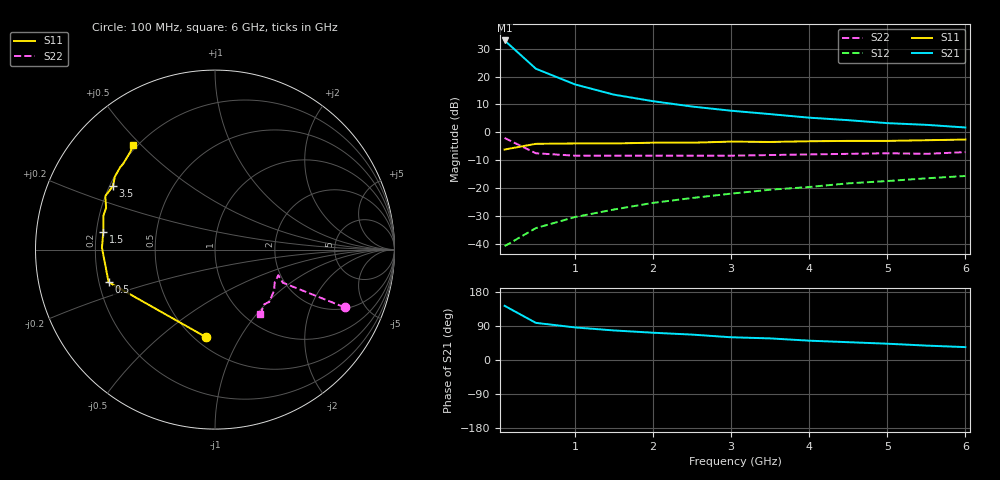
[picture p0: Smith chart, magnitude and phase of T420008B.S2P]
!AT-42000
!S-PARAMETERS at Vce=8V  Ic=35mA.  LAST UPDATED 07-21-92
# ghz s ma r 50
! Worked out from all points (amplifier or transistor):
!   13 points, 100 MHz to 6 GHz, reference 50 ohm
!   highest |S21| = 33.0 dB at 100 MHz (marker M1)
!   |S21| within 3 dB of that: start of sweep to 218.3 MHz
!   unconditionally stable (mu >= 1): 872.8 MHz to 4.032 GHz
!   at 1 GHz: K = 1.06, MAG = 22.4 dB, |S12| = -30.5 dB
!   at 3 GHz: K = 1.04, MAG = 13.6 dB, |S12| = -22.0 dB
!   at 6 GHz: K = 0.79, MSG = 8.7 dB, |S12| = -15.7 dB
!   S11 on the Smith chart (normalised r, x): 100 MHz: 0.57, -0.73; 500 MHz: 0.24, -0.14; 1.5 GHz: 0.23, +0.07; 3.5 GHz: 0.21, +0.27; 6 GHz: 0.18, +0.47
0.1  0.49 -96.0  44.61 143.0  0.009 65.0  0.79 -24.0
0.5  0.62 -163.0  13.87 98.0  0.019 58.0  0.42 -26.0
1  0.63 179.0  7.25 86.0  0.03 70.0  0.38 -22.0
1.5  0.63 171.0  4.74 78.0  0.041 76.0  0.38 -23.0
2  0.65 163.0  3.62 72.0  0.054 79.0  0.38 -25.0
2.5  0.65 159.0  2.9 67.0  0.066 82.0  0.38 -27.0
3  0.68 154.0  2.44 60.0  0.079 82.0  0.38 -29.0
3.5  0.67 148.0  2.12 57.0  0.093 84.0  0.39 -32.0
4  0.69 144.0  1.83 51.0  0.104 86.0  0.4 -34.0
4.5  0.7 139.0  1.65 47.0  0.121 86.0  0.41 -40.0
5  0.7 137.0  1.46 43.0  0.133 85.0  0.42 -44.0
5.5  0.72 131.0  1.36 38.0  0.149 86.0  0.41 -48.0
6  0.74 128.0  1.22 34.0  0.164 85.0  0.44 -55.0
